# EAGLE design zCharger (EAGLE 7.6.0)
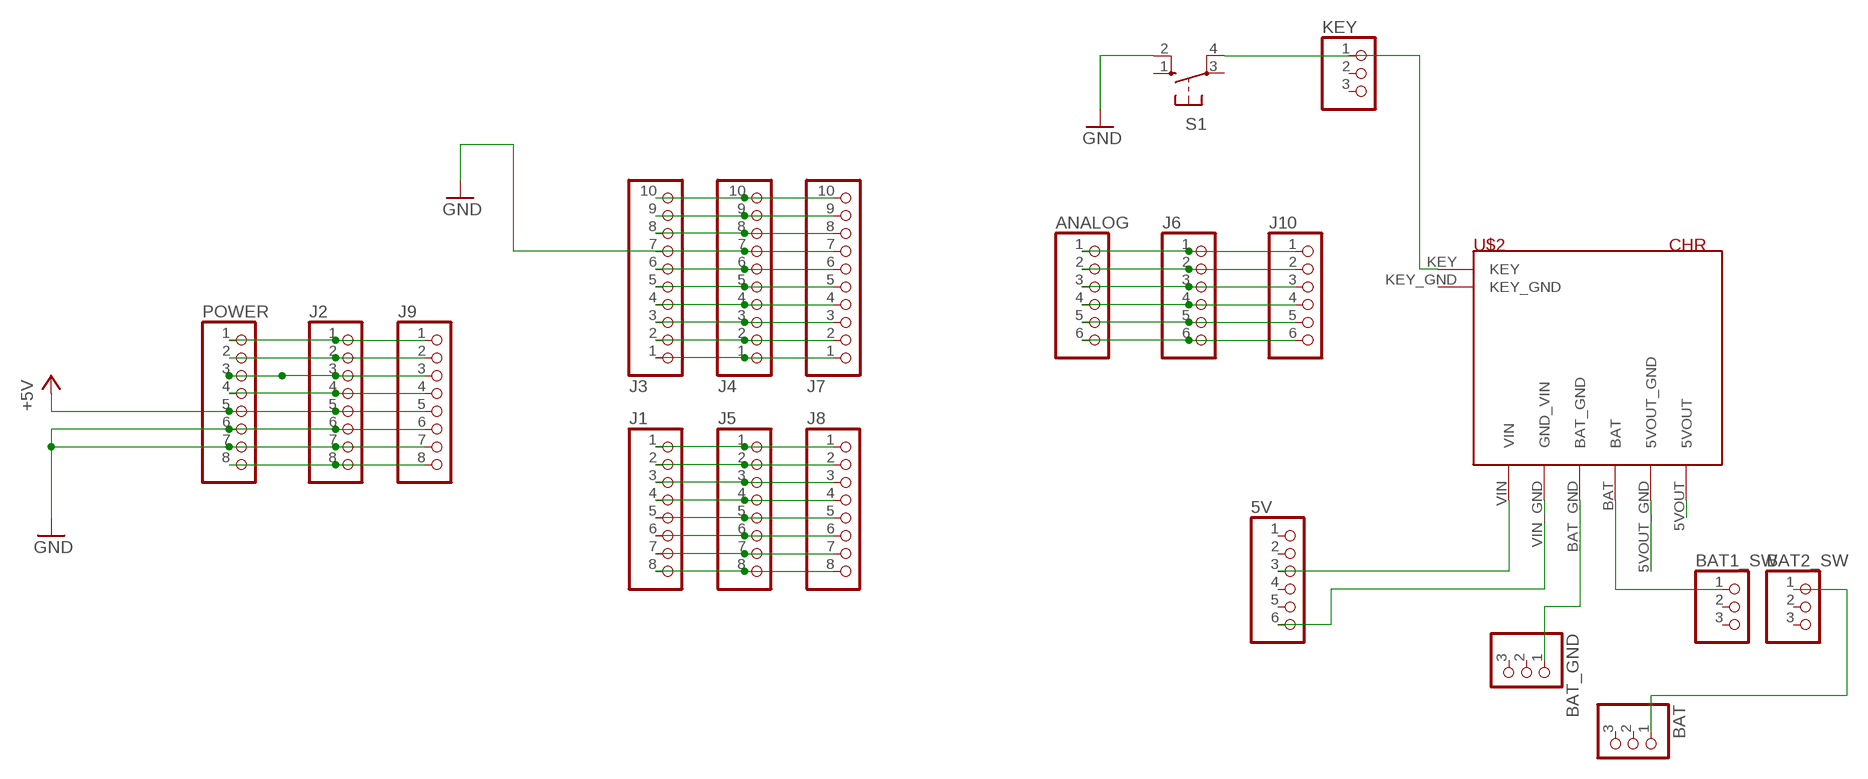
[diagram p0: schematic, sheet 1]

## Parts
5V  PINHD-1X6  [1X06]
ANALOG  PINHD-1X6  [1X06]
BAT  PINHD-1X3  [1X03]
BAT1_SW  PINHD-1X3  [1X03]
BAT2_SW  PINHD-1X3  [1X03]
BAT_GND  PINHD-1X3  [1X03]
J1  PINHD-1X8TH  [1X08-TH]
J2  PINHD-1X8TH  [1X08-TH]
J3  PINHD-1X10TH  [1X10-TH]
J4  PINHD-1X10TH  [1X10-TH]
J5  PINHD-1X8TH  [1X08-TH]
J6  PINHD-1X6  [1X06]
J7  PINHD-1X10TH  [1X10-TH]
J8  PINHD-1X8TH  [1X08-TH]
J9  PINHD-1X8TH  [1X08-TH]
J10  PINHD-1X6  [1X06]
KEY  PINHD-1X3  [1X03]
POWER  PINHD-1X8TH  [1X08-TH]
S1  10-XX  [B3F-10XX]
U$2  CHR  [CHARGER]

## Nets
+5V: J2.5 J9.5 POWER.5 U$2.5VOUT
+9V: J2.8 J9.8 POWER.8
GND: J2.6 J2.7 J3.7 J4.7 J7.7 J9.6 J9.7 POWER.6 POWER.7 S1.2(S1) U$2.5VOUT_GND
N$1: J3.6 J4.6 J7.6
N$2: J3.1 J4.1 J7.1
N$3: J3.4 J4.4 J7.4
N$4: J3.5 J4.5 J7.5
N$6: J3.2 J4.2 J7.2
N$7: J3.3 J4.3 J7.3
N$8: J1.1 J5.1 J8.1
N$9: J1.2 J5.2 J8.2
N$10: J1.3 J5.3 J8.3
N$11: J1.4 J5.4 J8.4
N$12: J1.5 J5.5 J8.5
N$13: J1.6 J5.6 J8.6
N$14: J1.7 J5.7 J8.7
N$15: J1.8 J5.8 J8.8
N$17: BAT_GND.1 U$2.BAT_GND
N$18: ANALOG.1 J6.1 J10.1
N$19: ANALOG.2 J6.2 J10.2
N$20: ANALOG.3 J6.3 J10.3
N$21: ANALOG.4 J6.4 J10.4
N$22: ANALOG.5 J6.5 J10.5
N$23: ANALOG.6 J6.6 J10.6
N$25: BAT1_SW.1 U$2.BAT
N$26: 5V.6 U$2.VIN_GND(GND_VIN)
N$27: 5V.3 U$2.VIN
N$28: KEY.1 S1.4(P1) U$2.KEY
N$31: J2.2 J9.2 POWER.2
N$32: J2.1 J9.1 POWER.1
N$68: BAT2_SW.1 BAT.1
N$141: J3.9 J4.9 J7.9
N$142: J3.10 J4.10 J7.10
N$222: J3.8 J4.8 J7.8
N$223: J2.4 J9.4 POWER.4
RESET: J2.3 J9.3 POWER.3
Unconnected: 5V.1 5V.2 5V.4 5V.5 BAT1_SW.2 BAT1_SW.3 BAT2_SW.2 BAT2_SW.3 BAT.2 BAT.3 BAT_GND.2 BAT_GND.3 KEY.2 KEY.3 S1.1(S) S1.3(P) U$2.KEY_GND

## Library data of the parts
5V = adafruit:PINHD-1X6: PIN HEADER
ANALOG J6 J10 = pinhead:PINHD-1X6: PIN HEADER
BAT BAT1_SW BAT2_SW BAT_GND KEY = adafruit:PINHD-1X3: PIN HEADER
J1 J2 J5 J8 J9 POWER = SmartPrj:PINHD-1X8: PIN HEADER
J3 J4 J7 = SmartPrj:PINHD-1X10: PIN HEADER
S1 = switch-omron:10-XX: OMRON SWITCH; MPN: B3F-1000; OC_FARNELL: 176432; OC_NEWARK: 36M3542
U$2 = charger:CHR

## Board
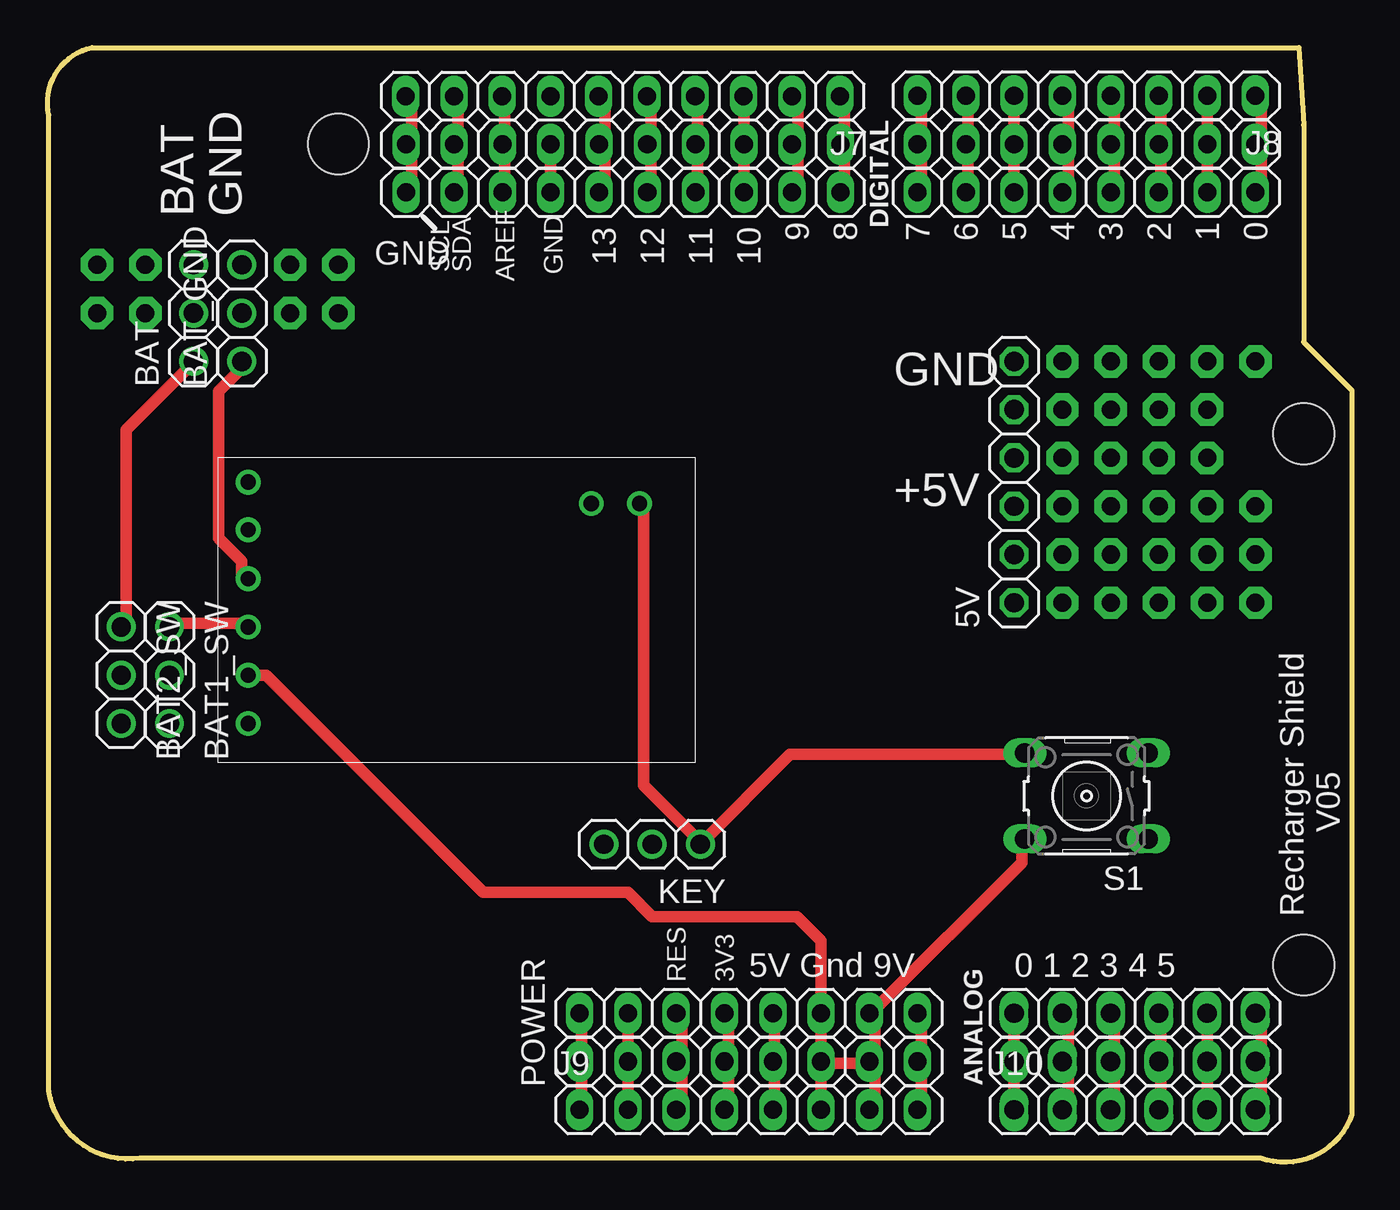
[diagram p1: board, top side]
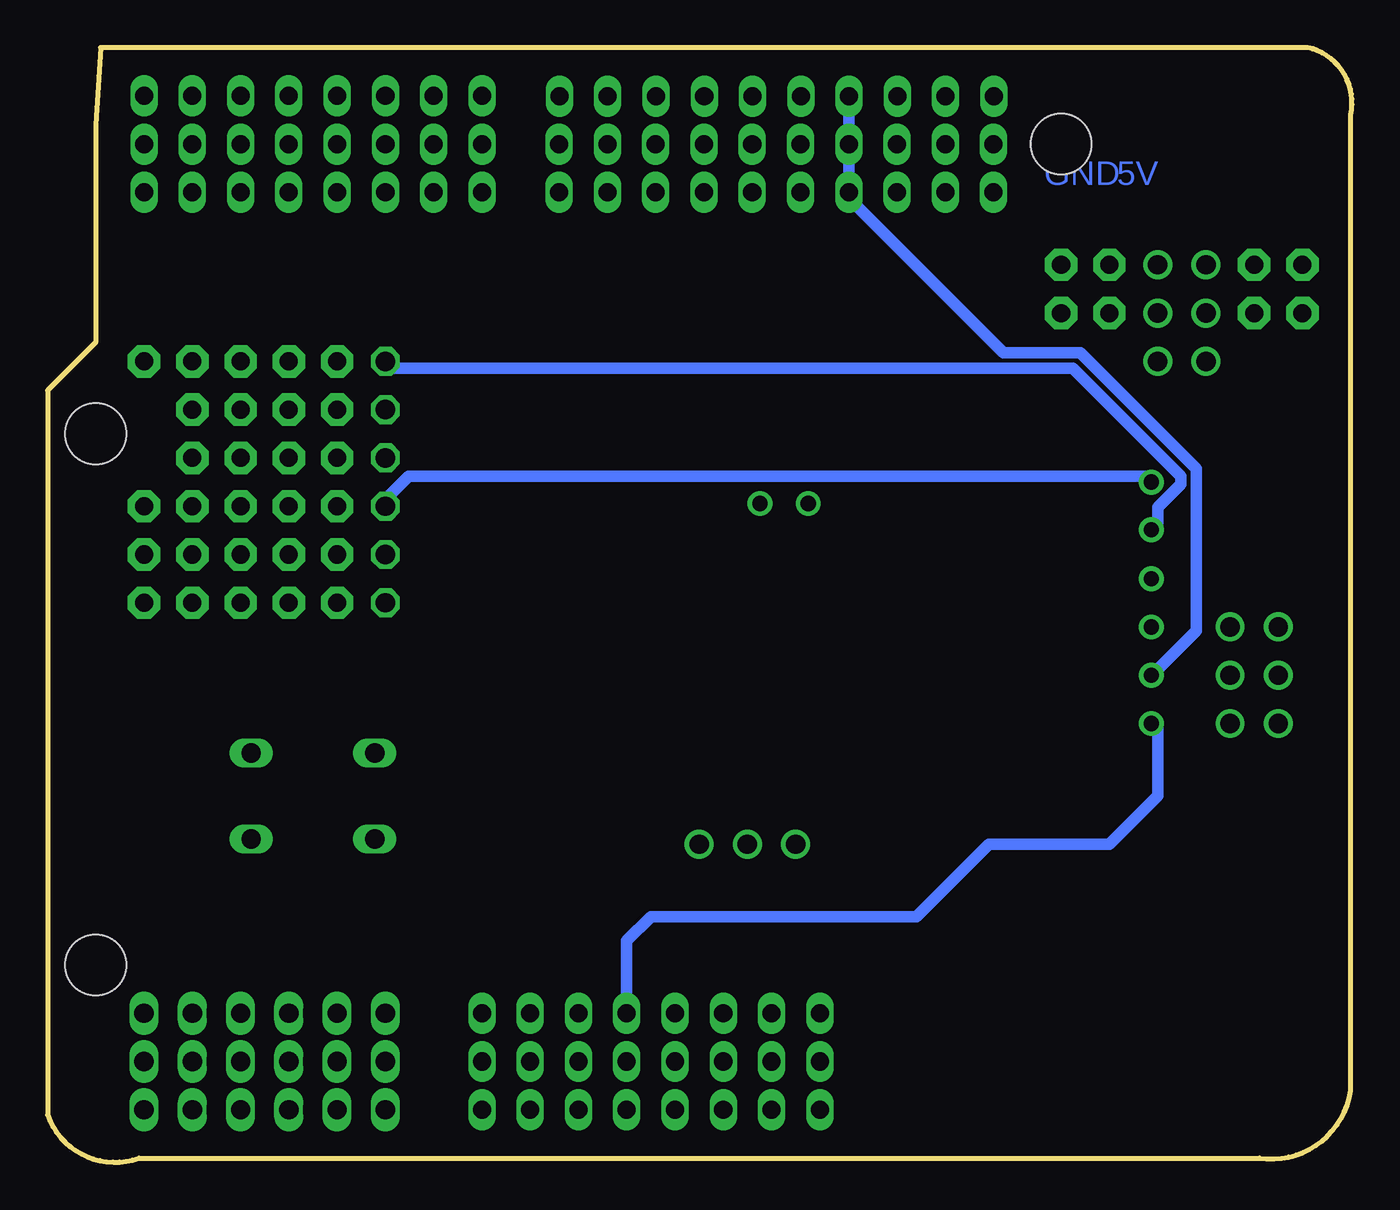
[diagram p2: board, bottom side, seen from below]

Size 68.65 x 58.64 mm. Coordinates in mm from the lower left corner, seen from the top.
Outline: 65.85,58.64 66.11,54.58 66.11,43.15 68.65,40.61 68.65,2.49 arc-90 63.84,0.22 4.88,0.22 arc-90 0.07,3.76 0.07,55.1 arc-90 2.34,58.64 65.85,58.64
Copper layers (1*16): Top 0.035mm / dielectric 1.5mm / Bottom 0.035mm
Design rules "default *": minimum track width 24mil, minimum drill 24mil, track to track 8mil, track to pad 8mil, pad to pad 8mil, via to via 8mil, smd to smd 8mil, copper to edge 40mil, drill to drill 8mil, minimum pad ring 10mil, minimum via ring 8mil, stop-mask expansion 2mil, vias tented up to drill 0mil, thermal gap 10mil
Holes 3.2 mm at 15.31,53.56 66.11,10.38 66.11,38.32

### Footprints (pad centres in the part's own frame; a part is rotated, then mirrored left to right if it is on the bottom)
1X06 = drill 1.016 octagon: 1 -6.35,0; 2 -3.81,0; 3 -1.27,0; 4 1.27,0; 5 3.81,0; 6 6.35,0
1X06' = drill 1.016 long: 1 -6.35,0; 2 -3.81,0; 3 -1.27,0; 4 1.27,0; 5 3.81,0; 6 6.35,0
1X03 = drill 1.016: 1 -2.54,0; 2 0,0; 3 2.54,0
1X08-TH = drill 0.95 pad 1.422 long: 1 -8.89,0; 2 -6.35,0; 3 -3.81,0; 4 -1.27,0; 5 1.27,0; 6 3.81,0; 7 6.35,0; 8 8.89,0
1X10-TH = drill 0.95 pad 1.422 long: 1 -11.43,0; 2 -8.89,0; 3 -6.35,0; 4 -3.81,0; 5 -1.27,0; 6 1.27,0; 7 3.81,0; 8 6.35,0; 9 8.89,0; 10 11.43,0
B3F-10XX = drill 1.016 long: 1 -3.251,2.261; 2 3.251,2.261; 3 -3.251,-2.261; 4 3.251,-2.261
CHARGER = drill 0.8: 5VOUT 13.97,1.6; 5VOUT_GND 11.43,1.6; BAT 8.89,1.6; BAT_GND 6.35,1.6; KEY 2.398,22.2; KEY_GND 2.398,19.66; VIN 1.27,1.6; VIN_GND 3.785,1.6

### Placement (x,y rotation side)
5V  50.87,35.78 90 top
ANALOG  [1X06']  57.22,5.3 0 top
BAT  7.69,44.67 90 top
BAT1_SW  6.42,25.62 270 top
BAT2_SW  3.88,25.62 270 top
BAT_GND  10.23,44.67 90 top
J1  54.68,53.56 180 top
J2  36.9,5.3 0 top
J3  30.29,53.56 180 top
J4  30.29,51.02 180 top
J5  54.68,51.02 180 top
J6  [1X06']  57.22,7.84 0 top
J7  30.28,56.08 180 top
J8  54.68,56.1 180 top
J9  36.9,2.76 0 top
J10  [1X06']  57.22,2.76 0 top
KEY  31.82,16.73 180 top
POWER  36.9,7.84 0 top
S1  54.68,19.27 180 top
U$2  8.96,37.05 270 top

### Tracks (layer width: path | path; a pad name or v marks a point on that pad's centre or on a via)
+5V
  Top 0.61: J9.5 38.27,2.76 38.27,5.2 J2.5 38.27,5.6 38.27,7.64 POWER.5
  Bottom 0.61: U$2.5VOUT 10.23,23.08 10.23,19.27 12.77,16.73 19.12,16.73 22.93,12.92 36.9,12.92 38.17,11.65 POWER.5
+9V
  Top 0.61: J9.8 45.99,2.76 45.99,5.2 J2.8 45.99,5.6 45.99,7.64 POWER.8
GND
  Top 0.61: 40.71,5.2 J9.6 | J9.7 43.55,2.76 43.55,5.2 J2.7 | J2.7 43.55,5.6 43.55,7.64 POWER.7 43.55,8.04 51.27,15.76 51.27,16.98 S1.2 | U$2.5VOUT_GND 11.5,25.62 22.93,14.19 30.55,14.19 31.82,12.92 39.44,12.92 40.71,11.65 POWER.6 J2.6 40.71,5.2 | 40.71,5.2 43.15,5.2 J2.7
  Bottom 0.61: J7.7 26.48,56 J3.7 J4.7 26.48,50.71 18.36,42.59 14.29,42.59 8.2,36.49 8.2,27.96 10.23,25.92 U$2.5VOUT_GND
N$1
  Top 0.61: 29.33,53.56 29.33,56 J7.6 | 29.33,53.56 29.33,51.12 J4.6 | 29.33,53.56 J3.6
N$2
  Top 0.61: 41.93,53.56 41.93,56 J7.1 | 41.93,53.56 41.93,51.12 J4.1 | 41.93,53.56 J3.1
N$3
  Top 0.61: 34.21,53.56 34.21,56 J7.4 | 34.21,53.56 34.21,51.12 J4.4 | 34.21,53.56 J3.4
N$4
  Top 0.61: 31.77,53.56 31.77,56 J7.5 | 31.77,53.56 31.77,51.12 J4.5 | 31.77,53.56 J3.5
N$5
  Top 0.61: 26.48,53.69 26.48,51.15
N$6
  Top 0.61: 39.49,53.56 39.49,56 J7.2 | 39.49,53.56 39.49,51.12 J4.2 | 39.49,53.56 J3.2
N$7
  Top 0.61: J7.3 36.64,56 J3.3 J4.3
N$8
  Top 0.61: 63.87,53.56 63.87,51.12 J5.1 | 63.87,53.56 63.87,56 J8.1 | 63.87,53.56 J1.1
N$9
  Top 0.61: J5.2 J1.2 J8.2
N$10
  Top 0.61: 58.59,53.56 58.59,51.12 J5.3 | 58.59,53.56 58.59,56 J8.3 | 58.59,53.56 J1.3
N$11
  Top 0.61: 56.15,53.56 56.15,51.12 J5.4 | 56.15,53.56 56.15,56 J8.4 | 56.15,53.56 J1.4
N$12
  Top 0.61: 53.71,53.56 53.71,51.12 J5.5 | 53.71,53.56 53.71,56 J8.5 | 53.71,53.56 J1.5
N$13
  Top 0.61: J5.6 J1.6 J8.6
N$14
  Top 0.61: 48.43,53.56 48.43,51.12 J5.7 | 48.43,53.56 48.43,56 J8.7 | 48.43,53.56 J1.7
N$15
  Top 0.61: 45.99,53.56 45.99,51.12 J5.8 | 45.99,53.56 45.99,56 J8.8 | 45.99,53.56 J1.8
N$16  (via drill 0.95 pad 1.7)
  Top 0.254: 61.1,37.05 v61.03,37.05
N$17
  Top 0.61: U$2.BAT_GND 10.23,30.8 10.23,31.61 9.01,32.83 9.01,40.55 10.23,41.77 BAT_GND.1
N$18
  Top 0.61: J10.1 ANALOG.1 J6.1
N$19
  Top 0.61: J10.2 53.71,2.76 53.71,5.2 ANALOG.2 53.71,5.6 53.71,7.64 J6.2
N$20
  Top 0.61: J10.3 56.15,2.76 56.15,5.2 ANALOG.3 56.15,5.6 56.15,7.64 J6.3
N$21
  Top 0.61: J10.4 58.59,2.76 58.59,5.2 ANALOG.4 58.59,5.6 58.59,7.64 J6.4
N$22
  Top 0.61: J10.5 ANALOG.5 J6.5
N$23
  Top 0.61: J10.6 63.87,2.76 63.87,5.2 ANALOG.6 63.87,5.6 63.87,7.64 J6.6
N$25
  Top 0.61: U$2.BAT 10.23,28.36 6.57,28.36 BAT1_SW.1
N$26
  Bottom 0.61: U$2.VIN_GND 10.23,33.65 10.23,34.46 9.01,35.68 9.01,36.08 14.7,41.77 50.87,41.77 5V.6
N$27
  Bottom 0.61: U$2.VIN 10.63,36.08 49.65,36.08 50.87,34.87 5V.3
N$28
  Top 0.61: U$2.KEY 31.36,34.46 31.36,19.83 34.21,16.98 KEY.1 39.08,21.45 51.27,21.45 S1.4
N$31
  Top 0.61: J9.2 J2.2 POWER.2
N$32
  Top 0.61: J9.1 28.11,2.76 28.11,5.2 J2.1 28.11,5.6 28.11,7.64 POWER.1
N$33  (via drill 0.95 pad 1.7)
  Top 0.254: 53.56,42.31 v53.41,42.13 53.33,42.31
N$34  (via drill 0.95 pad 1.7)
  other vias: 55.95,37.05
N$36  (via drill 0.95 pad 1.7)
  Top 0.254: 53.56,32.02 v53.41,31.97 53.56,31.79
N$37  (via drill 0.95 pad 1.7)
  other vias: 58.49,37.05
N$38  (via drill 0.95 pad 1.7)
  Top 0.254: 61.1,31.79 v61.03,31.97 61.1,32.02
N$39  (via drill 0.95 pad 1.7)
  Top 0.254: 63.62,32.02 v63.57,31.97 63.62,31.79
N$40  (via drill 0.95 pad 1.7)
  Top 0.254: 63.62,34.31 v63.57,34.51 63.39,34.53
N$41  (via drill 0.95 pad 1.7)
  Top 0.254: 63.62,29.51 v63.57,29.43
N$42  (via drill 0.95 pad 1.7)
  Top 0.254: 58.59,32.02 v58.49,31.97 58.59,31.79
N$43  (via drill 0.95 pad 1.7)
  Top 0.254: 58.59,34.53 v58.49,34.51 | 58.59,34.31 v58.49,34.51 | 58.36,34.53 v58.49,34.51
N$44  (via drill 0.95 pad 1.7)
  Top 0.254: 61.1,34.31 v61.03,34.51 | 61.1,34.53 v61.03,34.51 | 60.88,34.53 v61.03,34.51
N$45  (via drill 0.95 pad 1.7)
  Top 0.254: 61.1,29.51 v61.03,29.43
N$46  (via drill 0.95 pad 1.7)
  Top 0.254: 58.59,29.51 v58.49,29.43
N$47  (via drill 0.95 pad 1.7)
  Top 0.254: 56.07,29.51 v55.95,29.43
N$48  (via drill 0.95 pad 1.7)
  Top 0.254: 56.07,31.79 v55.95,31.97 56.07,32.02
N$49  (via drill 0.95 pad 1.7)
  Top 0.254: 56.07,34.31 v55.95,34.51 | 56.07,34.53 v55.95,34.51 | 55.85,34.53 v55.95,34.51
N$50  (via drill 0.95 pad 1.7)
  Top 0.254: 53.56,34.53 v53.41,34.51 53.56,34.31
N$51  (via drill 0.95 pad 1.7)
  Top 0.254: 53.56,29.51 v53.41,29.43
N$52  (via drill 0.95 pad 1.7)
  Top 0.254: 15.16,47.34 v15.31,47.21 15.38,47.11
N$53  (via drill 0.95 pad 1.7)
  Top 0.254: 15.38,44.82 v15.31,44.67 15.38,44.59
N$54  (via drill 0.95 pad 1.7)
  Top 0.254: 12.87,47.34 v12.77,47.21 12.87,47.11
N$55  (via drill 0.95 pad 1.7)
  Top 0.254: 12.87,44.82 v12.77,44.67
N$56  (via drill 0.95 pad 1.7)
  Top 0.254: 5.33,44.82 v5.15,44.67 5.1,44.82
N$57  (via drill 0.95 pad 1.7)
  Top 0.254: 5.1,47.34 v5.15,47.21
N$58  (via drill 0.95 pad 1.7)
  Top 0.254: 2.81,44.82 v2.61,44.67 2.58,44.82
N$59  (via drill 0.95 pad 1.7)
  Top 0.254: 63.39,42.31 v63.57,42.13
N$60  (via drill 0.95 pad 1.7)
  Top 0.254: 58.59,42.31 v58.49,42.13 58.36,42.31
N$61  (via drill 0.95 pad 1.7)
  Top 0.254: 61.1,42.31 v61.03,42.13 61.1,42.08
N$62  (via drill 0.95 pad 1.7)
  Top 0.254: 56.07,42.31 v55.95,42.13 55.85,42.31
N$63  (via drill 0.95 pad 1.7)
  Top 0.254: 53.56,39.56 v53.41,39.59
N$64  (via drill 0.95 pad 1.7)
  Top 0.254: 56.07,39.56 v55.95,39.59 55.85,39.56
N$65  (via drill 0.95 pad 1.7)
  other vias: 53.41,37.05
N$66  (via drill 0.95 pad 1.7)
  Top 0.254: 58.59,39.56 v58.49,39.59 58.36,39.56
N$67  (via drill 0.95 pad 1.7)
  Top 0.254: 61.1,39.56 v61.03,39.59 | 61.1,39.79 v61.03,39.59 | 60.88,39.56 v61.03,39.59
N$68
  Top 0.61: BAT2_SW.1 4.13,28.36 4.13,38.52 7.38,41.77 BAT.1
N$141
  Top 0.61: 21.61,53.56 21.61,56 J7.9 | 21.61,53.56 21.61,51.12 J4.9 | 21.61,53.56 J3.9
N$142
  Top 0.61: 19.17,53.56 19.17,56 J7.10 | 19.17,53.56 19.17,51.12 J4.10 | 19.17,53.56 J3.10
N$203  (via drill 0.95 pad 1.7)
  Top 0.254: 2.58,47.11 v2.61,47.21 2.81,47.34
N$222
  Top 0.61: 24.05,53.56 24.05,56 J7.8 | 24.05,53.56 24.05,51.12 J4.8 | 24.05,53.56 J3.8
N$223
  Top 0.61: J9.4 35.83,2.76 35.83,5.2 J2.4 35.83,5.6 35.83,7.64 POWER.4
RESET
  Top 0.61: J9.3 33.39,2.76 33.39,5.2 J2.3 33.39,5.6 33.39,7.64 POWER.3

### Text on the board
Bottom: 5V | GND
tPlace: BAT | GND | 9 | 8 | 7 | 6 | 5 | 4 | 3 | 2 | 1 | 0 | GND | 13 | 12 | 11 | 10 | GND | +5V | V05 | Recharger Shield
tNames: DIGITAL | AREF | SCL | SDA | GND | RES | 3V3 | 5V Gnd 9V | 0 1 2 3 4 5
bStop: DIGITAL | SDA | AREF | SCL | GND | 13 | 12 | 11 | 9 | 8 | 7 | 6 | 5 | 4 | 3 | 2 | 1 | 0 | 10 | IOREF | RST | 3.3V | 5V | GND | GND | VIN | ANALOG | 0 | 1 | 2 | 3 | 4 | 5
